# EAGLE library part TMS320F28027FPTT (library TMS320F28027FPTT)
Piccolo 32-bit MCU with 60 MHz, 64 KB Flash, InstaSPIN-FOC Source: Datasheet
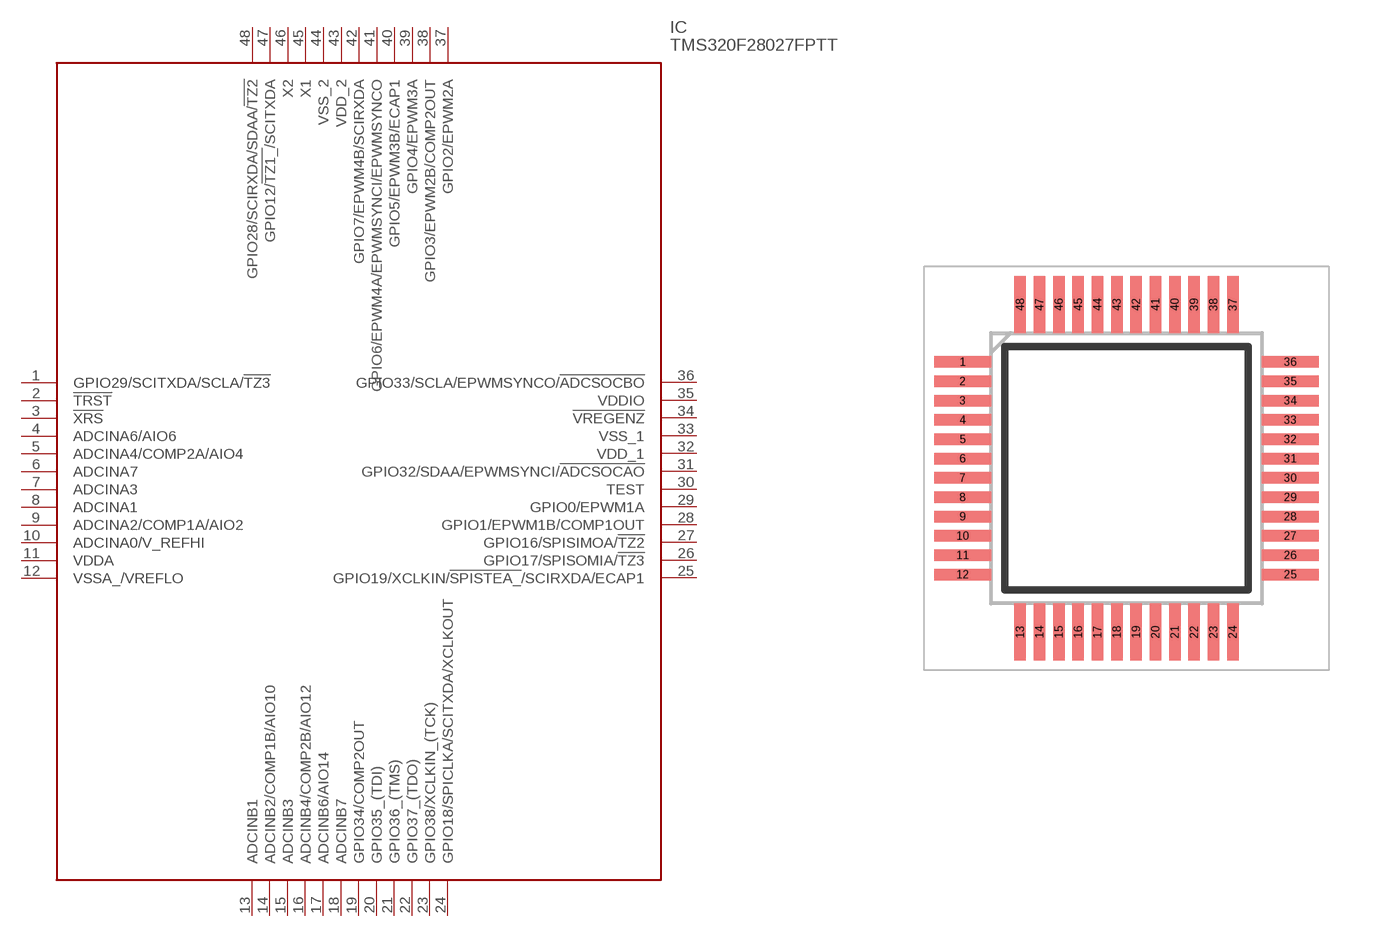
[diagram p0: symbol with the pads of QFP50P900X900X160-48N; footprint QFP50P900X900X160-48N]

Designator prefix IC

## TMS320F28027FPTT (Description: Piccolo 32-bit MCU with 60 MHz, 64 KB Flash, InstaSPIN-FOC; Height: 1.6mm; Manufacturer_Name: Texas Instruments; Manufacturer_Part_Number: TMS320F28027FPTT; Mouser_Part_Number: 595-TMS320F28027FPTT; Mouser_Price-Stock: https://www.mouser.com/Search/Refine.aspx?Keyword=595-TMS320F28027FPTT)  [QFP50P900X900X160-48N]
1  GPIO29/SCITXDA/SCLA/!TZ3
2  !TRST
3  !XRS
4  ADCINA6/AIO6
5  ADCINA4/COMP2A/AIO4
6  ADCINA7
7  ADCINA3
8  ADCINA1
9  ADCINA2/COMP1A/AIO2
10  ADCINA0/V_REFHI
11  VDDA
12  VSSA_/VREFLO
13  ADCINB1
14  ADCINB2/COMP1B/AIO10
15  ADCINB3
16  ADCINB4/COMP2B/AIO12
17  ADCINB6/AIO14
18  ADCINB7
19  GPIO34/COMP2OUT
20  GPIO35_(TDI)
21  GPIO36_(TMS)
22  GPIO37_(TDO)
23  GPIO38/XCLKIN_(TCK)
24  GPIO18/SPICLKA/SCITXDA/XCLKOUT
25  GPIO19/XCLKIN/!SPISTEA_!/SCIRXDA/ECAP1
26  GPIO17/SPISOMIA/!TZ3
27  GPIO16/SPISIMOA/!TZ2
28  GPIO1/EPWM1B/COMP1OUT
29  GPIO0/EPWM1A
30  TEST
31  GPIO32/SDAA/EPWMSYNCI/!ADCSOCAO
32  VDD_1
33  VSS_1
34  !VREGENZ
35  VDDIO
36  GPIO33/SCLA/EPWMSYNCO/!ADCSOCBO
37  GPIO2/EPWM2A
38  GPIO3/EPWM2B/COMP2OUT
39  GPIO4/EPWM3A
40  GPIO5/EPWM3B/ECAP1
41  GPIO6/EPWM4A/EPWMSYNCI/EPWMSYNCO
42  GPIO7/EPWM4B/SCIRXDA
43  VDD_2
44  VSS_2
45  X1
46  X2
47  GPIO12/!TZ1_!/SCITXDA
48  GPIO28/SCIRXDA/SDAA/!TZ2

## Footprint QFP50P900X900X160-48N (pad centres in mm)
TMS320F28027FPTT
smd 1.475 x 0.3: 1 -4.238,2.75; 2 -4.238,2.25; 3 -4.238,1.75; 4 -4.238,1.25; 5 -4.238,0.75; 6 -4.238,0.25; 7 -4.238,-0.25; 8 -4.238,-0.75; 9 -4.238,-1.25; 10 -4.238,-1.75; 11 -4.238,-2.25; 12 -4.238,-2.75; 25 4.238,-2.75; 26 4.238,-2.25; 27 4.238,-1.75; 28 4.238,-1.25; 29 4.238,-0.75; 30 4.238,-0.25; 31 4.238,0.25; 32 4.238,0.75; 33 4.238,1.25; 34 4.238,1.75; 35 4.238,2.25; 36 4.238,2.75
smd 0.3 x 1.475: 13 -2.75,-4.238; 14 -2.25,-4.238; 15 -1.75,-4.238; 16 -1.25,-4.238; 17 -0.75,-4.238; 18 -0.25,-4.238; 19 0.25,-4.238; 20 0.75,-4.238; 21 1.25,-4.238; 22 1.75,-4.238; 23 2.25,-4.238; 24 2.75,-4.238; 37 2.75,4.238; 38 2.25,4.238; 39 1.75,4.238; 40 1.25,4.238; 41 0.75,4.238; 42 0.25,4.238; 43 -0.25,4.238; 44 -0.75,4.238; 45 -1.25,4.238; 46 -1.75,4.238; 47 -2.25,4.238; 48 -2.75,4.238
